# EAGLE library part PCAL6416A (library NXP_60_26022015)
Low-voltage translating 16-bit I2C-bus/SMBus I/O expander with interrupt output, reset, and configuration registers The PCAL6416A is a 16-bit general-purpose I/O expander that provides remote I/O expansion for most microcontroller families via the I2C-bus interface. NXP I/O expanders provide a simple solution when additional I/Os are needed while keeping interconnections to a minimum, for example, in battery-powered mobile applications for interfacing to sensors, push buttons, keypad, etc. In addition to providing a flexible set of GPIOs, it simplifies interconnection of a processor running at one voltage level to I/O devices operating at a different (usually higher) voltage level. The PCAL6416A has built-in level shifting feature that makes these devices extremely flexible in mixed signal environments where communication between incompatible I/O voltages is required. Its wide VDD range of 1.65 V to 5.5 V on the dual power rail allows seamless communications with next-generation low voltage microprocessors and microcontrollers on the interface side (SDA/SCL) and peripherals at a higher voltage on the port side. There are two supply voltages for PCAL6416A: VDD(I2C-bus) and VDD(P). VDD(I2C-bus) provides the supply voltage for the interface at the master side (for example, a microcontroller) and the VDD(P) provides the supply for core circuits and Port P. The bidirectional voltage level translation in the PCAL6416A is provided through VDD(I2C-bus). VDD(I2C-bus) should be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
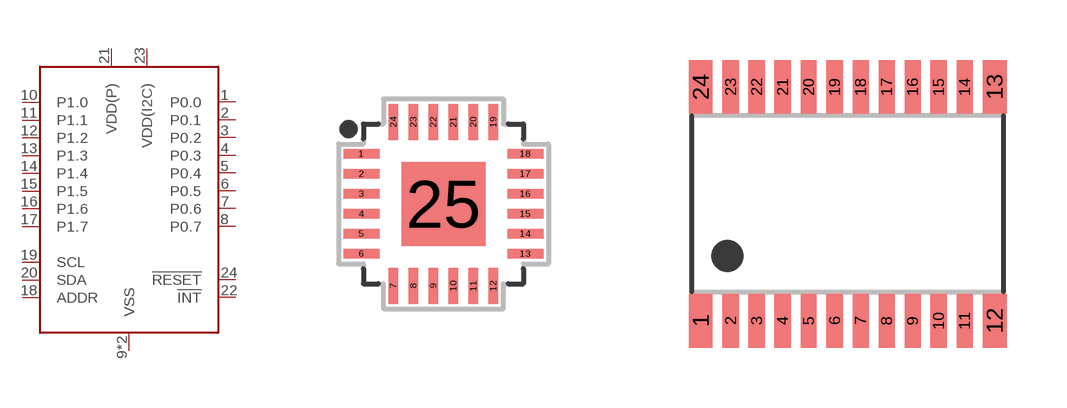
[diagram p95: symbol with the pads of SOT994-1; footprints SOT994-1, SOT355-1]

Designator prefix -

## PCAL6416AHF  [SOT994-1]
1  P0.0
2  P0.1
3  P0.2
4  P0.3
5  P0.4
6  P0.5
7  P0.6
8  P0.7
9  VSS
10  P1.0
11  P1.1
12  P1.2
13  P1.3
14  P1.4
15  P1.5
16  P1.6
17  P1.7
18  ADDR  in
19  SCL
20  SDA
21  VDD(P)  pwr
22  !INT!  out
23  VDD(I2C)  pwr
24  !RESET!  in
25  VSS

## PCAL6416APW  [SOT355-1]
1  !INT!  out
2  VDD(I2C)  pwr
3  !RESET!  in
4  P0.0
5  P0.1
6  P0.2
7  P0.3
8  P0.4
9  P0.5
10  P0.6
11  P0.7
12  VSS
13  P1.0
14  P1.1
15  P1.2
16  P1.3
17  P1.4
18  P1.5
19  P1.6
20  P1.7
21  ADDR  in
22  SCL
23  SDA
24  VDD(P)  pwr

## PCAL6416AEV  [SOT1199-1]
A1  P0.0
A2  !RESET!  in
A3  !INT!  out
A4  SDA
A5  SCL
B1  P0.2
B3  VDD(I2C)  pwr
B4  VDD(P)  pwr
B5  ADDR  in
C1  P0.3
C2  P0.4
C3  P0.1
C4  P1.7
C5  P1.6
D1  P0.5
D2  P0.7
D3  P1.2
D4  P1.4
D5  P1.5
E1  P0.6
E2  VSS
E3  P1.0
E4  P1.1
E5  P1.3

## Footprint SOT994-1 (pad centres in mm)
SOT994-1 HWQFN24: plastic thermal enhanced very very thin quad flat package; no leads; 24 terminals; body 4 x 4 x 0.75 mm JEDEC: IEC: -- JEITA: --
smd 0.9 x 0.24: 1 -2.05,1.25; 2 -2.05,0.75; 3 -2.05,0.25; 4 -2.05,-0.25; 5 -2.05,-0.75; 6 -2.05,-1.25; 13 2.05,-1.25; 14 2.05,-0.75; 15 2.05,-0.25; 16 2.05,0.25; 17 2.05,0.75; 18 2.05,1.25
smd 0.24 x 0.9: 7 -1.25,-2.05; 8 -0.75,-2.05; 9 -0.25,-2.05; 10 0.25,-2.05; 11 0.75,-2.05; 12 1.25,-2.05; 19 1.25,2.05; 20 0.75,2.05; 21 0.25,2.05; 22 -0.25,2.05; 23 -0.75,2.05; 24 -1.25,2.05
smd 2.1 x 2.1: 25 0,0

## Footprint SOT355-1 (pad centres in mm)
SOT355-1 TSSOP24: plastic thin shrink small outline package; 24 leads; body width 4.4 mm JEDEC: MO-153 IEC: -- JEITA: --
smd 0.6 x 1.35: 1 -3.675,-2.925; 12 3.675,-2.925; 13 3.675,2.925; 24 -3.675,2.925
smd 0.4 x 1.35: 2 -2.925,-2.925; 3 -2.275,-2.925; 4 -1.625,-2.925; 5 -0.975,-2.925; 6 -0.325,-2.925; 7 0.325,-2.925; 8 0.975,-2.925; 9 1.625,-2.925; 10 2.275,-2.925; 11 2.925,-2.925; 14 2.925,2.925; 15 2.275,2.925; 16 1.625,2.925; 17 0.975,2.925; 18 0.325,2.925; 19 -0.325,2.925; 20 -0.975,2.925; 21 -1.625,2.925; 22 -2.275,2.925; 23 -2.925,2.925

## Footprint SOT1199-1 (pad centres in mm)
SOT1199-1 VFBGA24: plastic very thin fine-pitch ball grid array package; 24 balls; body 3 x 3 x 0.65 mm JEDEC: -- IEC: -- JEITA: --
smd 0.255 x 0.255: A1 -1,1; A2 -0.5,1; A3 0,1; A4 0.5,1; A5 1,1; B1 -1,0.5; B3 0,0.5; B4 0.5,0.5; B5 1,0.5; C1 -1,0; C2 -0.5,0; C3 0,0; C4 0.5,0; C5 1,0; D1 -1,-0.5; D2 -0.5,-0.5; D3 0,-0.5; D4 0.5,-0.5; D5 1,-0.5; E1 -1,-1; E2 -0.5,-1; E3 0,-1; E4 0.5,-1; E5 1,-1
